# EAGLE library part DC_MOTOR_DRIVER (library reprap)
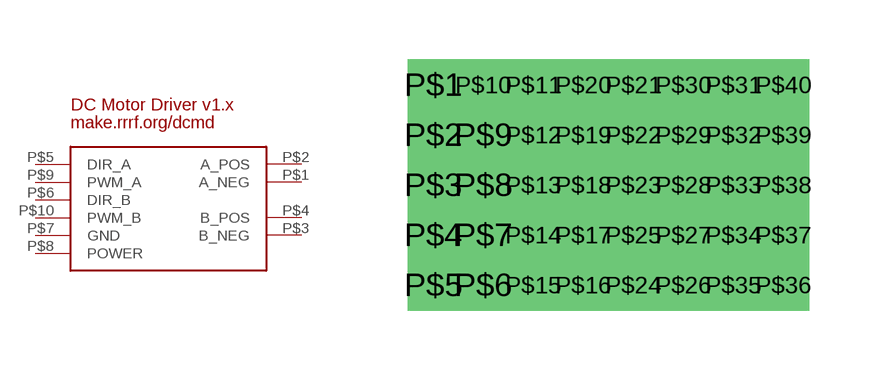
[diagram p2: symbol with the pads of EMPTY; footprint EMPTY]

Designator prefix -

## DC_MOTOR_DRIVER  [EMPTY]
P$1  A_NEG
P$2  A_POS
P$3  B_NEG
P$4  B_POS
P$5  DIR_A
P$6  DIR_B
P$7  GND
P$8  POWER
P$9  PWM_A
P$10  PWM_B

## Footprint EMPTY (pad centres in mm)
drill 0.8 square: P$1 -1.27,5.08; P$2 -1.27,3.81; P$3 -1.27,2.54; P$4 -1.27,1.27; P$5 -1.27,0; P$6 0,0; P$7 0,1.27; P$8 0,2.54; P$9 0,3.81; P$10 0,5.08; P$11 1.27,5.08; P$12 1.27,3.81; P$13 1.27,2.54; P$14 1.27,1.27; P$15 1.27,0; P$16 2.54,0; P$17 2.54,1.27; P$18 2.54,2.54; P$19 2.54,3.81; P$20 2.54,5.08; P$21 3.81,5.08; P$22 3.81,3.81; P$23 3.81,2.54; P$24 3.81,0; P$25 3.81,1.27; P$26 5.08,0; P$27 5.08,1.27; P$28 5.08,2.54; P$29 5.08,3.81; P$30 5.08,5.08; P$31 6.35,5.08; P$32 6.35,3.81; P$33 6.35,2.54; P$34 6.35,1.27; P$35 6.35,0; P$36 7.62,0; P$37 7.62,1.27; P$38 7.62,2.54; P$39 7.62,3.81; P$40 7.62,5.08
